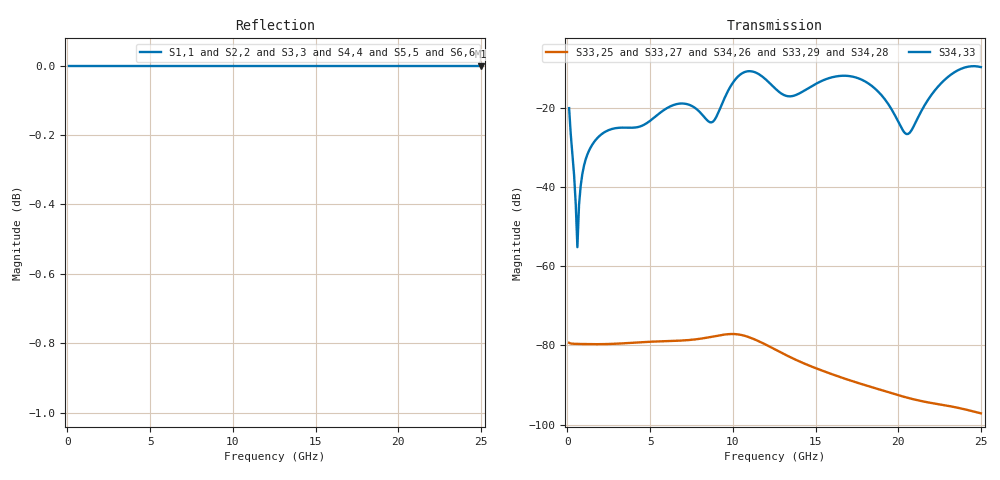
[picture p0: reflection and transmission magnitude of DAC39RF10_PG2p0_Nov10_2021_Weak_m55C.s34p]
! Touchstone Ver. 1.0
! Number of ports is 34
# Hz	S	RI	R	50.000000
! SCATTERING PARAMETERS  :
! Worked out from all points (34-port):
!   250 points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, 100 MHz to 25 GHz, reference 50 ohm
!   strongest paths, dB at 100 MHz, 6.3 GHz, 12.6 GHz, 18.8 GHz, 25 GHz:
!     S34,33: -20.2, -19.6, -15.4, -16.0, -9.8
!     S33,25: -79.3, -78.9, -81.1, -91.0, -97.1
!     S33,27: -79.3, -78.9, -81.1, -91.1, -97.2
!     S34,26: -79.4, -78.9, -81.2, -91.0, -97.2
!     S33,29: -79.3, -78.9, -81.2, -91.1, -97.3
!     S34,28: -79.4, -78.9, -81.2, -91.1, -97.2
!   lowest |S11| = 0.0 dB at 25 GHz (marker M1)
!   |S11| at or under -10 dB: nowhere
